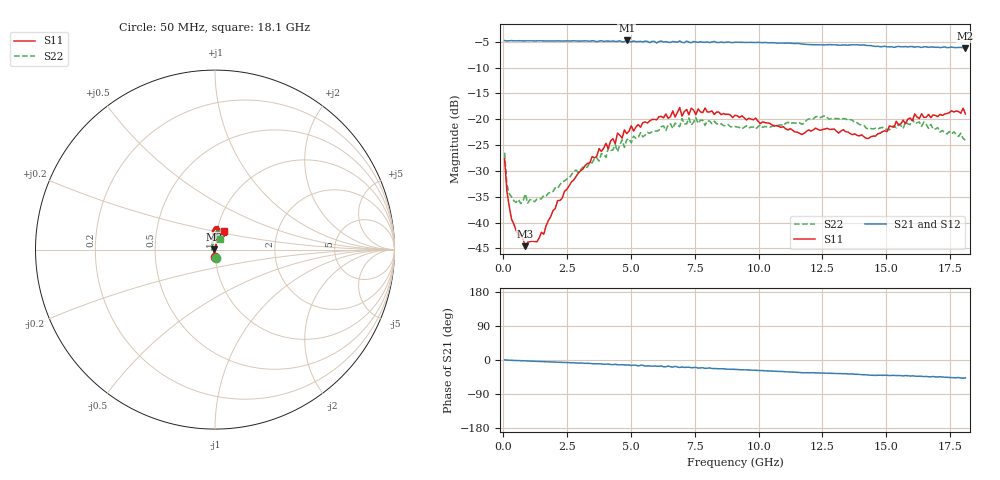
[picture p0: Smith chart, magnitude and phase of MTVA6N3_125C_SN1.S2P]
! Network Analyzer HP8720D.06.14 Serial No. US36140669
!  5 Jul 2005  10:10:11
! Frequency  S11  S21  S12  S22
# HZ  S  DB R 50
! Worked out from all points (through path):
!   201 points, 50 MHz to 18.1 GHz, reference 50 ohm
!   highest |S21| = -4.77 dB at 4.833 GHz (marker M1); lowest = -6.3 dB at 18.1 GHz (marker M2)
!   group delay of S21, straight-line fit = 7.43 ps
!   lowest |S11| = -44.6 dB at 862.2 MHz (marker M3), VSWR 1.01, Z = 49.4 + j0.101 ohm
!   |S11| at or under -10 dB: start of sweep to end of sweep
!   |S22| runs from -36.3 to -19.3 dB; largest |S21 - S12| = 0.02
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5e7  -27.67 -90.8  -4.78 0.3  -4.81 0.4  -26.49 -83.7
1.4025e8  -33.99 -103.2  -4.86 -0.3  -4.83 -0.2  -32.66 -121.0
2.305e8  -36.83 -112.6  -4.83 -0.5  -4.82 -0.5  -34.37 -136.9
6.8175e8  -42.29 -167.4  -4.83 -1.8  -4.85 -1.8  -36.33 -173.0
8.6225e8  -44.57 170.1  -4.83 -2.2  -4.85 -2.2  -34.48 -179.6
9.525e8  -43.81 167.2  -4.84 -2.4  -4.84 -2.5  -36.24 174.6
1.58425e9  -42.26 110.0  -4.85 -4.3  -4.85 -4.2  -34.75 149.1
2.12575e9  -35.76 83.6  -4.84 -5.9  -4.86 -5.8  -33.36 124.3
3.1185e9  -29.67 79.4  -4.87 -8.2  -4.89 -8.5  -29.23 117.8
3.75025e9  -25.70 76.9  -4.88 -10.0  -4.91 -9.7  -28.11 107.0
4.382e9  -24.70 75.9  -4.95 -11.3  -4.92 -12.3  -24.89 102.9
4.47225e9  -22.70 72.7  -4.94 -12.3  -4.88 -11.7  -26.28 104.8
4.83325e9  -22.79 82.3  -4.77 -12.9  -4.87 -13.6  -23.98 91.1
6.09675e9  -19.50 78.6  -4.98 -16.6  -4.91 -16.6  -22.14 88.0
6.909e9  -17.75 84.0  -4.87 -19.6  -4.98 -18.6  -21.44 81.6
7.54075e9  -19.12 83.0  -5.07 -19.5  -4.94 -21.4  -19.70 86.1
9.075e9  -19.24 94.9  -5.12 -24.7  -5.09 -24.8  -21.43 75.8
1.21435e10  -22.05 89.2  -5.58 -33.5  -5.54 -33.8  -19.93 77.0
1.43095e10  -23.72 64.3  -5.76 -39.9  -5.73 -40.2  -21.88 81.3
1.512175e10  -21.31 61.9  -6.01 -41.1  -5.91 -40.9  -22.06 84.3
1.602425e10  -20.31 55.1  -5.95 -41.8  -6.07 -43.4  -19.98 69.6
1.81e10  -18.98 64.1  -6.31 -47.3  -6.37 -48.2  -24.07 65.6
